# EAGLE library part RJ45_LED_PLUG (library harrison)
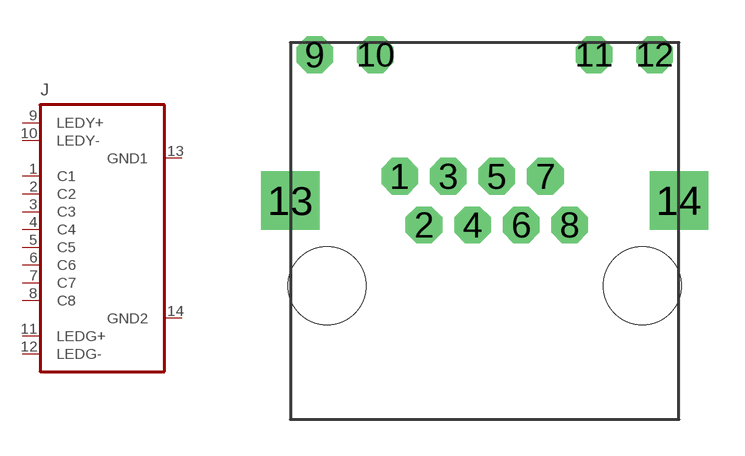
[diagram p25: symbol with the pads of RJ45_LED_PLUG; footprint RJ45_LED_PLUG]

Designator prefix J

## RJ45_LED_PLUG  [RJ45_LED_PLUG]
1  C1  pas
2  C2  pas
3  C3  pas
4  C4  pas
5  C5  pas
6  C6  pas
7  C7  pas
8  C8  pas
9  LEDY+  pas
10  LEDY-  pas
11  LEDG+  pas
12  LEDG-  pas
13  GND1  pwr
14  GND2  pwr

## Footprint RJ45_LED_PLUG (pad centres in mm)
drill 1 octagon: 1 4.5,10; 2 5.5,8; 3 6.5,10; 4 7.5,8; 5 8.5,10; 6 9.5,8; 7 10.5,10; 8 11.5,8; 9 1,15; 10 3.5,15; 11 12.5,15; 12 15,15
drill 1.6 square: 13 0,9; 14 16,9
hole 3.2 at 1.5,5.5
hole 3.2 at 14.5,5.5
